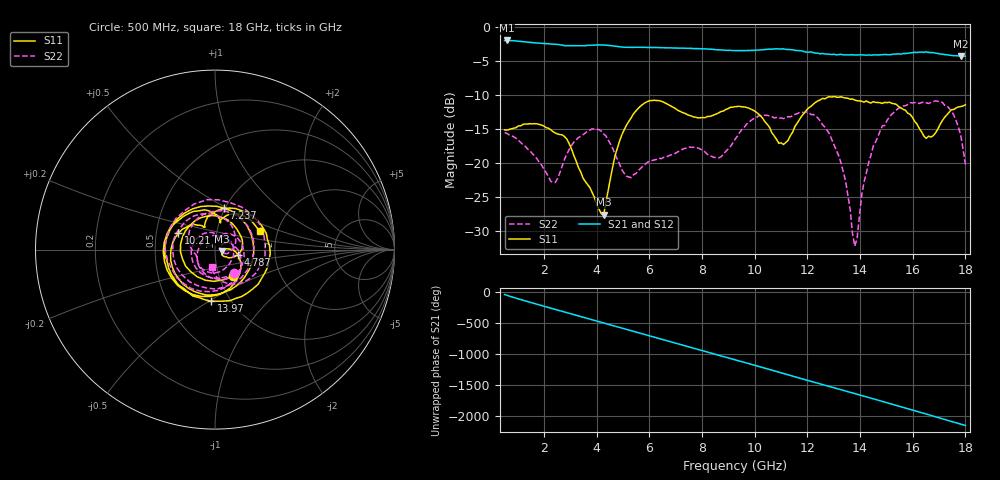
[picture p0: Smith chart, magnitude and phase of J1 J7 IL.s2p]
!Agilent Technologies,N5230A,MY45001360,A.07.50.67
!Agilent N5230A: A.07.50.67
!Date: Tuesday, April 16, 2024 16:34:23
!Correction: S11(Full 2 Port(1,2))
!S21(Full 2 Port(1,2))
!S12(Full 2 Port(1,2))
!S22(Full 2 Port(1,2))
!S2P File: Measurements: S11, S21, S12, S22:
# Hz S  dB  R 50
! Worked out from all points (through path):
!   201 points, 500 MHz to 18 GHz, reference 50 ohm
!   highest |S21| = -1.93 dB at 587.5 MHz (marker M1); lowest = -4.3 dB at 17.82 GHz (marker M2)
!   group delay of S21, straight-line fit = 333 ps
!   lowest |S11| = -27.6 dB at 4.263 GHz (marker M3), VSWR 1.09, Z = 54.2 - j1.03 ohm
!   |S11| at or under -10 dB: start of sweep to end of sweep
!   |S22| runs from -32.2 to -10.8 dB; largest |S21 - S12| = 0.0096
!   S11 on the Smith chart (normalised r, x): 500 MHz: 1.16, -0.35; 4.787 GHz: 1.29, -0.07; 7.237 GHz: 0.99, +0.48; 10.21 GHz: 0.65, +0.13; 13.97 GHz: 0.81, -0.51; 18 GHz: 1.61, +0.36
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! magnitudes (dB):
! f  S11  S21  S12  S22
! 500 MHz  -15.1  -1.9  -1.9  -15.5
! 587.5 MHz  -15.2  -1.9  -1.9  -15.6
! 2.425 GHz  -15.6  -2.5  -2.5  -22.9
! 3.475 GHz  -22.2  -2.7  -2.7  -15.8
! 4.263 GHz  -27.6  -2.6  -2.6  -15.7
! 4.787 GHz  -17.8  -2.8  -2.8  -19.5
! 5.312 GHz  -13.3  -2.9  -2.9  -22.2
! 6.362 GHz  -10.8  -3.0  -3.0  -19.3
! 7.237 GHz  -12.5  -3.1  -3.1  -18.0
! 9.25 GHz  -11.7  -3.4  -3.4  -16.5
! 10.21 GHz  -13.0  -3.3  -3.3  -13.0
! 11.09 GHz  -17.3  -3.2  -3.2  -13.4
! 12.22 GHz  -11.3  -3.7  -3.7  -12.8
! 13.19 GHz  -10.3  -4.0  -4.0  -18.9
! 13.8 GHz  -10.7  -4.1  -4.1  -32.2
! 13.97 GHz  -10.8  -4.1  -4.1  -27.9
! 14.5 GHz  -10.9  -4.1  -4.0  -17.5
! 15.11 GHz  -11.0  -4.0  -4.0  -13.2
! 16.51 GHz  -16.4  -3.6  -3.6  -11.1
! 17.3 GHz  -12.9  -4.0  -4.1  -11.5
! 17.82 GHz  -11.7  -4.3  -4.2  -15.9
! 18 GHz  -11.4  -4.2  -4.3  -20.2
